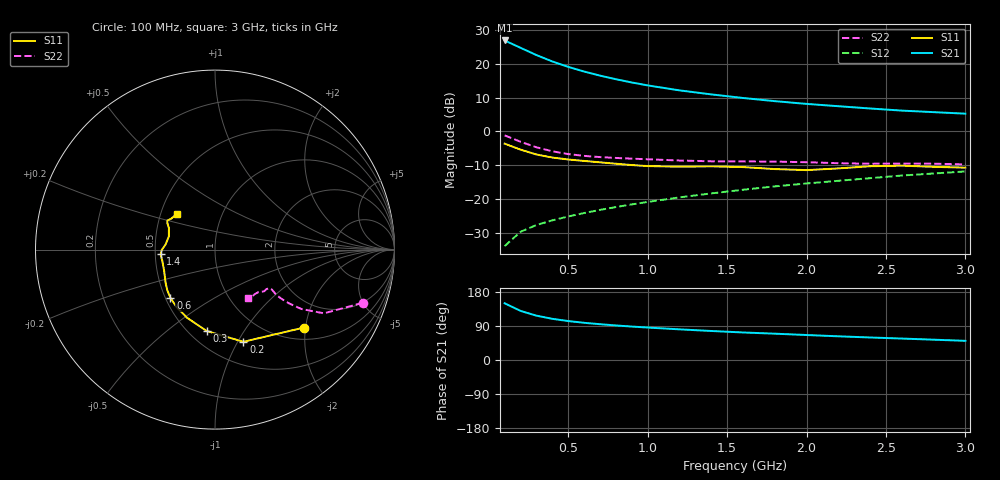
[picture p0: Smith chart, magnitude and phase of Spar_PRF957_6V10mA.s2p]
! Filename:  PRF957N.S2P  Version:  3.0
! NXP part #:  PRF957  Date:  Nov 1998
! Bias condition:  Vce=6V, Ic=10mA
#  MHz  S  MA  R 50
! Freq  S11  S21  S12  S22
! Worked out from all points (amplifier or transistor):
!   20 points, 100 MHz to 3 GHz, reference 50 ohm
!   highest |S21| = 26.9 dB at 100 MHz (marker M1)
!   |S21| within 3 dB of that: start of sweep to 238.7 MHz
!   unconditionally stable (mu >= 1): 1.073 GHz to end of sweep
!   at 400 MHz: K = 0.70, MSG = 23.5 dB, |S12| = -26.3 dB
!   at 1.2 GHz: K = 1.02, MAG = 15.0 dB, |S12| = -19.5 dB
!   at 3 GHz: K = 1.04, MAG = 7.4 dB, |S12| = -11.8 dB
!   lowest NFmin = 1.22 dB at 500 MHz
!   S11 on the Smith chart (normalised r, x): 100 MHz: 1.28, -1.96; 200 MHz: 0.73, -1.06; 300 MHz: 0.61, -0.70; 600 MHz: 0.53, -0.33; 1.4 GHz: 0.53, -0.03; 3 GHz: 0.61, +0.26
100  0.6595 -41.2  22.2 149.7  0.02003 71.8  0.875 -19.8
200  0.5374 -72.9  17.3 129.6  0.03267 63.2  0.7029 -30.4
300  0.4558 -95.8  13.49 117.0  0.04117 60.8  0.583 -34.5
400  0.4106 -112.2  10.85 108.7  0.04825 61.2  0.508 -36.0
500  0.3842 -124.1  9.021 102.8  0.05506 62.7  0.4626 -36.5
600  0.3657 -132.8  7.699 98.2  0.06193 64.3  0.4345 -36.5
700  0.3489 -139.7  6.702 94.4  0.06891 65.7  0.417 -36.2
800  0.3327 -145.7  5.927 91.2  0.0759 67.1  0.4051 -35.8
900  0.3177 -151.6  5.301 88.3  0.08309 68.3  0.3955 -35.4
1000  0.307 -157.4  4.799 85.7  0.09046 69.3  0.3868 -35.1
1200  0.3003 -168.0  4.051 80.9  0.1055 70.7  0.3711 -35.5
1400  0.304 -175.0  3.533 76.6  0.1209 71.5  0.3614 -37.4
1600  0.2968 -179.6  3.126 72.7  0.1369 72.2  0.3594 -39.5
1800  0.2772 174.2  2.806 69.4  0.1537 72.5  0.3577 -40.7
2000  0.2675 164.2  2.555 65.9  0.1696 72.7  0.3501 -41.9
2200  0.2833 155.0  2.361 62.5  0.1858 72.6  0.3386 -44.4
2400  0.3053 150.6  2.185 59.4  0.2032 72.3  0.3324 -48.1
2600  0.3114 148.6  2.032 56.6  0.2224 71.7  0.3338 -51.5
2800  0.2991 144.9  1.929 53.6  0.2384 71.6  0.3331 -53.6
3000  0.2909 137.2  1.831 50.6  0.2558 71.3  0.3248 -55.7
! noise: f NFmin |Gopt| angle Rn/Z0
500  1.22  0.16  28  0.16
800  1.4  0.19  81  0.16
900  1.51  0.21  75  0.16
1000  1.5  0.19  81  0.23
1500  1.5  0.29  126  0.16
2000  1.86  0.27  -165  0.15
